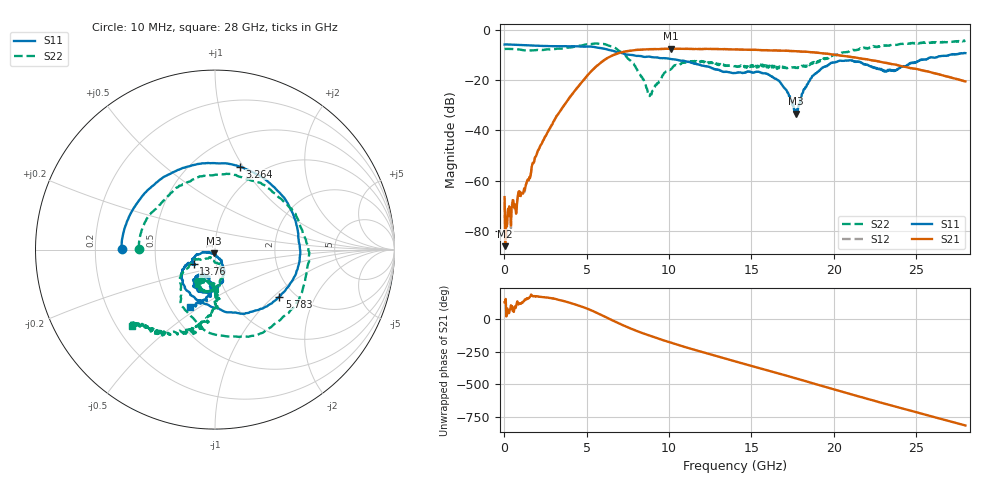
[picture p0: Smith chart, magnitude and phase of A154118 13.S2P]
!  2-Port S-parameters saved by WinCal
! VAR MeasName=S-Parameters (CALIBRATED_DATA) read from VNA (N5230A)
! VAR MeasDate=2015-9-10 14:35:20
! VAR NAME=A154118 13
! VAR FILENAME=A154118 13.S2P
! VAR DATE=2015-9-10 14:35:20
! VAR PHYS_PORTS=1,2
# Hz S DB R 50
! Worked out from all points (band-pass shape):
!   801 points, 10 MHz to 28 GHz, reference 50 ohm
!   highest |S21| = -7.38 dB at 10.12 GHz (marker M1); lowest = -86.2 dB at 44.99 MHz (marker M2)
!   |S21| within 3 dB of the highest: 6.461 GHz to 20.77 GHz (14.3 GHz wide, 105 % of centre)
!   lowest |S11| = -33.3 dB at 17.71 GHz (marker M3), VSWR 1.04, Z = 49.2 - j2 ohm
!   |S11| at or under -10 dB: 7.847 GHz to 26.98 GHz (19.13 GHz wide, 110 % of centre)
!   |S22| runs from -26.3 to -4.1 dB; largest |S21 - S12| = 0.0069
!   S11 on the Smith chart (normalised r, x): 10 MHz: 0.32, +0.00; 3.264 GHz: 0.80, +0.97; 5.783 GHz: 1.67, -1.09; 13.76 GHz: 0.78, -0.13; 28 GHz: 0.63, -0.46
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1e7  -5.69 179.6  -66.63 127.1  -68.83 -81.9  -7.48 179.8
4.49875e7  -5.67 178.6  -86.22 128.3  -79.01 71.7  -7.46 178.7
2.549125e8  -5.68 171.7  -74.20 42.4  -74.79 68.4  -7.44 172.1
1.1296e9  -5.97 145.1  -65.25 131.6  -64.85 129.7  -7.93 146.1
2.004288e9  -6.19 118.3  -48.61 172.1  -48.64 172.0  -7.84 122.3
3.263838e9  -6.33 73.5  -33.45 146.4  -33.43 146.5  -7.30 78.0
4.698325e9  -6.51 12.0  -20.76 93.3  -20.71 93.1  -6.06 12.4
5.782938e9  -7.05 -36.2  -13.28 36.1  -13.24 35.8  -5.43 -47.2
6.412712e9  -7.99 -60.5  -10.53 -2.2  -10.50 -2.6  -6.29 -83.6
7.182438e9  -9.20 -82.1  -8.73 -47.4  -8.70 -47.4  -9.00 -122.2
8.791862e9  -10.50 -110.2  -7.58 -127.0  -7.52 -127.5  -25.84 -118.1
9.351662e9  -10.96 -119.4  -7.54 -151.0  -7.48 -151.4  -21.08 -70.4
1.012139e10  -11.48 -129.1  -7.38 177.9  -7.36 177.4  -15.49 -78.6
1.211568e10  -14.20 -150.3  -7.46 103.8  -7.44 103.2  -12.81 -109.9
1.376009e10  -16.92 -146.3  -7.63 44.6  -7.62 44.0  -14.13 -120.4
1.4005e10  -17.11 -146.5  -7.66 36.2  -7.64 35.7  -14.36 -119.9
1.65241e10  -19.56 -164.7  -8.04 -51.3  -8.04 -51.5  -15.01 -111.3
1.771368e10  -33.27 -110.5  -8.37 -94.1  -8.37 -94.4  -15.07 -102.0
1.869332e10  -18.32 -65.3  -8.76 -129.7  -8.79 -130.0  -12.85 -89.0
2.040771e10  -12.12 -98.8  -10.09 168.1  -10.08 167.5  -9.15 -92.7
2.334666e10  -16.01 -110.8  -13.21 64.8  -13.23 64.2  -6.12 -112.2
2.8e10  -9.11 -113.1  -20.42 -92.6  -20.46 -92.5  -4.06 -137.4
